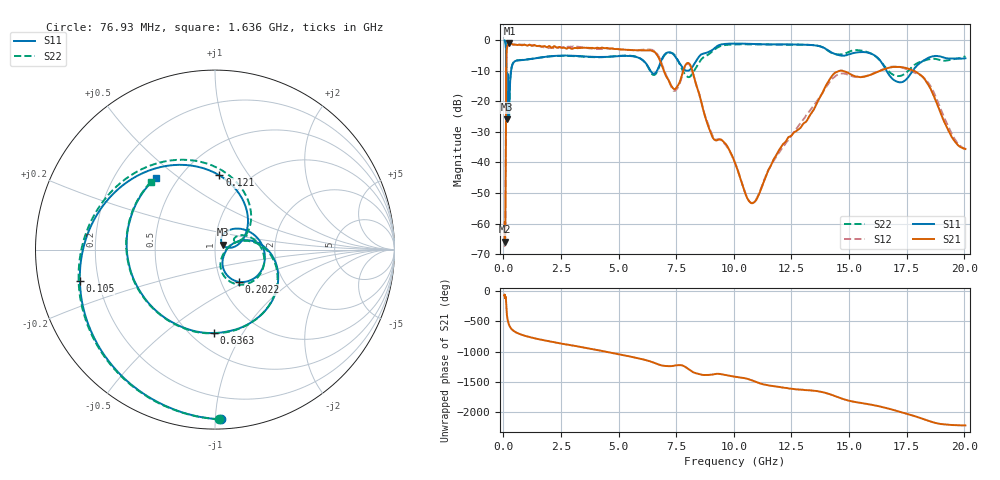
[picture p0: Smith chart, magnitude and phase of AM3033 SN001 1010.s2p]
# Hz S DB R 50
!freq MagS11 AngS11 MagS21 AngS21 MagS12 AngS12 MagS22 AngS22
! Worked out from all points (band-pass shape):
!   1601 points, 50 MHz to 20.05 GHz, reference 50 ohm
!   highest |S21| = -0.97 dB at 257 MHz (marker M1); lowest = -65.9 dB at 57.01 MHz (marker M2)
!   |S21| within 3 dB of the highest: 134.3 MHz to 6.574 GHz (6.44 GHz wide, 192 % of centre)
!   lowest |S11| = -25.9 dB at 137.5 MHz (marker M3), VSWR 1.11, Z = 54.4 + j3.04 ohm
!   |S11| at or under -10 dB: 124 MHz to 331.3 MHz (207.2 MHz wide, 91 % of centre); 6.379 GHz to 6.667 GHz (288.6 MHz wide, 4.42 % of centre); 16.62 GHz to 17.77 GHz (1.147 GHz wide, 6.67 % of centre)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
!   |S22| runs from -25.6 to -0.1 dB; largest |S21 - S12| = 0.064
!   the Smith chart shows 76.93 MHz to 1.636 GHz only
!   S11 on the Smith chart (normalised r, x): 76.93 MHz: 0.06, -1.03; 105 MHz: 0.13, -0.11; 121 MHz: 0.74, +0.74; 202.2 MHz: 1.21, -0.46; 636.3 MHz: 0.64, -0.76; 1.636 GHz: 0.38, +0.42
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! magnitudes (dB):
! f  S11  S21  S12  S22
! 50 MHz  -0.1  -59.6  -65.5  -0.1
! 57.01 MHz  -0.2  -65.9  -65.7  -0.2
! 76.93 MHz  -0.5  -62.6  -62.7  -0.5
! 89.03 MHz  -0.9  -56.6  -56.7  -0.9
! 105 MHz  -2.2  -31.5  -31.5  -2.3
! 121 MHz  -7.6  -10.3  -10.3  -7.1
! 135.9 MHz  -25.3  -3.7  -3.7  -18.2
! 137.5 MHz  -25.9  -3.5  -3.5  -18.5
! 202.2 MHz  -13.0  -1.4  -1.5  -13.2
! 257 MHz  -21.2  -1.0  -1.0  -21.3
! 369.6 MHz  -8.5  -1.3  -1.3  -8.5
! 636.3 MHz  -6.7  -1.6  -1.6  -6.6
! 1.005 GHz  -6.4  -1.8  -1.5  -6.4
! 1.636 GHz  -5.7  -2.1  -2.1  -5.7
! 2.722 GHz  -5.1  -2.8  -2.4  -5.2
! 6.396 GHz  -10.2  -3.4  -3.1  -10.5
! 7.402 GHz  -4.9  -16.0  -16.6  -4.7
! 8.129 GHz  -9.5  -8.5  -8.7  -11.7
! 10.77 GHz  -1.3  -53.3  -53.2  -1.4
! 14.58 GHz  -5.0  -10.1  -11.1  -4.7
! 17.78 GHz  -9.8  -10.0  -10.5  -8.5
! 20.05 GHz  -6.0  -35.6  -35.5  -5.3
